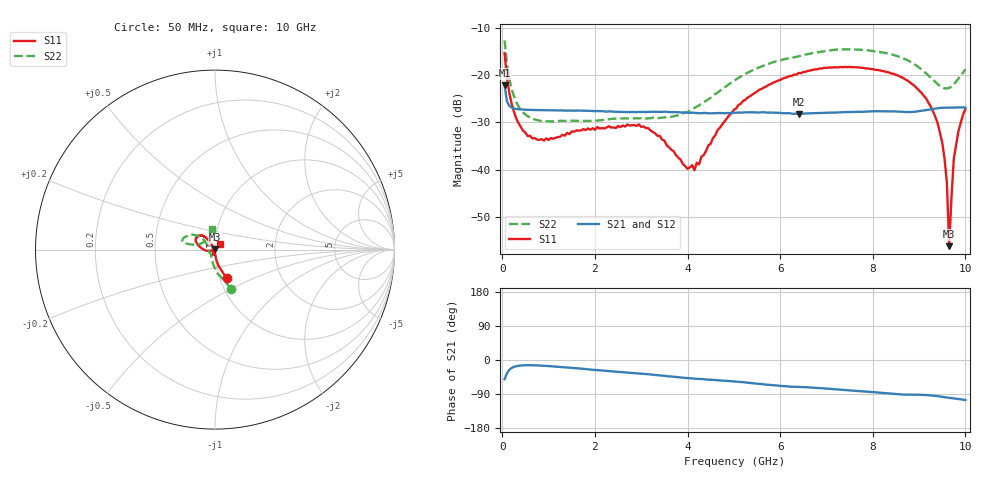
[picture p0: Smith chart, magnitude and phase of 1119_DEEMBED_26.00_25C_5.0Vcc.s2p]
!Hittite Microwave Corp.
!Digital Attenuator/PhaseShifter Rev 1.4.0
!Filename: C:\DATA\DATA\1119_DEEMBED_26.00_25C_5.0Vcc.s2p
!VNA ID: Agilent Technologies,N5224A,MY51441122,A.10.45.03
!Device type:
!2 Port Calibration.
!Temp(C): 25
!Lot Number:
!Serial Number:
!Operator:
!Misc:
!Attenuator:  26.000
# GHZ S DB R 50.0
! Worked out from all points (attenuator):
!   200 points, 50 MHz to 10 GHz, reference 50 ohm
!   highest |S21| = -22.07 dB at 50 MHz (marker M1); lowest = -28.2 dB at 6.4 GHz (marker M2)
!   lowest |S11| = -56.3 dB at 9.65 GHz (marker M3), VSWR 1.00, Z = 49.9 + j0.121 ohm
!   |S11| at or under -10 dB: start of sweep to end of sweep
!   |S22| runs from -29.8 to -12.6 dB; largest |S21 - S12| = 0.00013
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0.05  -15.26 -67.9  -22.07 -50.7  -22.07 -50.8  -12.56 -67.3
0.1  -20.46 -77.4  -25.50 -34.9  -25.49 -34.9  -17.51 -83.9
0.2  -25.95 -83.4  -26.82 -21.1  -26.83 -21.1  -22.79 -100.5
0.55  -32.89 -89.6  -27.31 -13.8  -27.31 -13.7  -28.67 -126.4
1  -33.72 -97.1  -27.40 -16.0  -27.41 -16.1  -29.73 -137.1
1.75  -31.41 -108.5  -27.49 -23.4  -27.50 -23.4  -29.66 -140.7
2.95  -30.41 -108.9  -27.75 -35.3  -27.76 -35.4  -29.12 -159.9
3.4  -32.84 -118.3  -27.74 -40.5  -27.74 -40.5  -29.03 -173.5
4.15  -40.16 170.4  -27.95 -49.4  -27.96 -49.4  -26.92 156.1
4.65  -31.60 124.9  -27.99 -53.4  -28.01 -53.5  -23.63 142.0
5.05  -27.03 122.0  -27.92 -57.0  -27.94 -57.1  -20.83 138.8
6.4  -19.46 132.5  -28.17 -71.1  -28.19 -71.1  -15.93 150.0
6.7  -18.83 137.1  -28.03 -73.0  -28.04 -73.0  -15.24 153.9
8.35  -19.36 160.8  -27.64 -88.5  -27.64 -88.5  -15.40 168.1
8.999999  -23.16 176.9  -27.61 -91.7  -27.61 -91.7  -18.33 167.3
9.400001  -30.08 -167.0  -26.97 -95.3  -26.99 -95.4  -21.83 153.7
9.5  -34.29 -166.0  -26.89 -97.3  -26.89 -97.3  -22.59 143.9
9.6  -42.74 -167.0  -26.85 -99.0  -26.86 -99.0  -22.76 132.3
9.65  -56.30 127.7  -26.83 -99.8  -26.85 -99.8  -22.64 126.1
9.75  -37.74 43.5  -26.82 -101.3  -26.83 -101.4  -21.90 114.2
9.85  -31.84 45.6  -26.80 -103.0  -26.81 -103.0  -20.67 106.1
10  -27.15 49.1  -26.84 -105.5  -26.84 -105.5  -18.66 98.5
